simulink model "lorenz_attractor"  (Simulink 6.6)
settings: Solver=ode23  SolverMode=SingleTasking  StartTime=0.0  StopTime=100  FixedStep=0.01  RelTol=1e-3
InitFcn:
  | lorenz_attractor_ini
StopFcn:
  | lorenz_attractor_plot
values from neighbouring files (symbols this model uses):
  beta = 1    [lorenz_attractor_ini.m]
  rho = 26.5    [lorenz_attractor_ini.m]
  sigma = 3    [lorenz_attractor_ini.m]
libraries: simulink x1

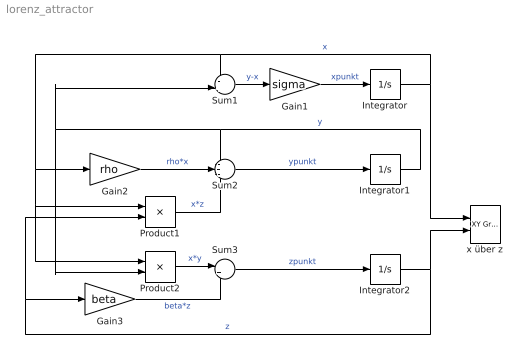
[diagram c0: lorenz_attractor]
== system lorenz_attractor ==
  Gain1 : Gain  Gain=sigma
  Gain2 : Gain  Gain=rho
  Gain3 : Gain  Gain=beta
  Integrator : Integrator  InitialCondition=5
  Integrator1 : Integrator  InitialCondition=5
  Integrator2 : Integrator  InitialCondition=5
  Product1 : Product
  Product2 : Product
  Sum1 : Sum  Inputs=-+|
  Sum2 : Sum  Inputs=-+-
  Sum3 : Sum  Inputs=|+-
  x über z : simulink/Sinks/XY Graph  SystemSampleTime=-1  xmin=-15  xmax=15  ymin=0  ymax=50  st=-1
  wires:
  Sum1/1 -> Gain1/1  "y-x"
  Gain1/1 -> Integrator/1  "xpunkt"
  Integrator/1 -> x über z/1, Sum1/1, Gain2/1, Product1/1, Product2/1  "x"
  Integrator2/1 -> x über z/2, Product1/2, Gain3/1  "z"
  Product1/1 -> Sum2/3  "x*z"
  Sum2/1 -> Integrator1/1  "ypunkt"
  Gain2/1 -> Sum2/2  "rho*x"
  Product2/1 -> Sum3/1  "x*y"
  Gain3/1 -> Sum3/2  "beta*z"
  Integrator1/1 -> Sum2/1, Product2/2, Sum1/2  "y"
  Sum3/1 -> Integrator2/1  "zpunkt"
